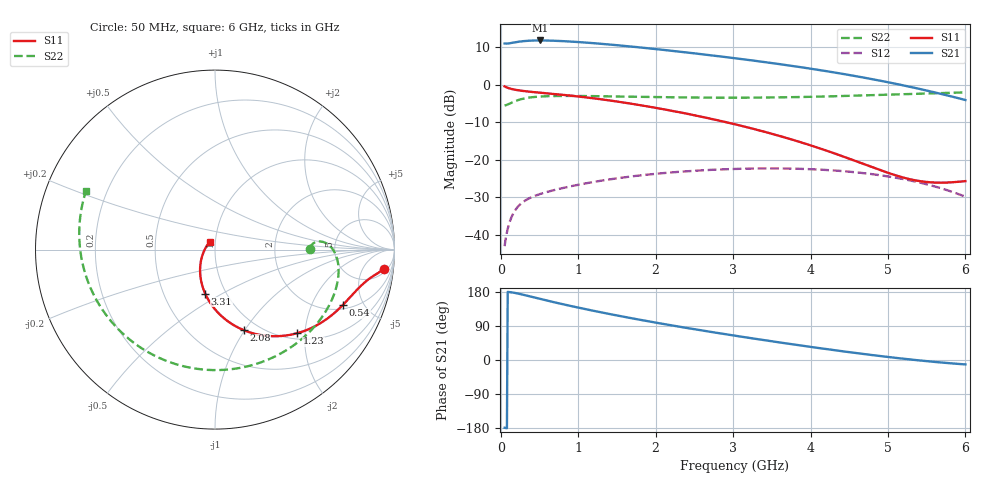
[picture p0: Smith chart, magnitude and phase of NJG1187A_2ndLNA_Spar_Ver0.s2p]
! Created Wed Mar 10 19:50:59 2021
# hz S ma R 50
! 2 Port Network Data from SP11.SP block
! freq  magS11  angS11  magS21  angS21  magS12  angS12  magS22  angS22
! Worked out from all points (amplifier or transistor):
!   596 points, 50 MHz to 6 GHz, reference 50 ohm
!   highest |S21| = 11.8 dB at 510 MHz (marker M1)
!   |S21| within 3 dB of that: start of sweep to 2.316 GHz
!   unconditionally stable (mu >= 1): start of sweep to end of sweep
!   at 1.04 GHz: K = 1.07, MAG = 17.2 dB, |S12| = -26.5 dB
!   at 3.03 GHz: K = 1.55, MAG = 10.4 dB, |S12| = -22.4 dB
!   at 6 GHz: K = 9.29, MAG = 0.2 dB, |S12| = -29.8 dB
!   lowest NFmin = 1.65 dB at 950 MHz
!   S11 on the Smith chart (normalised r, x): 50 MHz: 7, -15; 540 MHz: 2.24, -3.47; 1.23 GHz: 1.12, -1.82; 2.08 GHz: 0.85, -0.99; 3.31 GHz: 0.80, -0.42; 6 GHz: 0.94, +0.08
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5e7  0.9488 -6.5  3.533 -178.8  0.007091 81.8  0.5277 0.5
1.2e8  0.8874 -9.8  3.565 179.1  0.01537 68.4  0.563 4.3
2e8  0.8516 -12.6  3.686 176.4  0.02231 58.2  0.6113 3.8
3.4e8  0.8134 -17.0  3.833 169.7  0.02971 47.9  0.6668 -1.4
5.1e8  0.7816 -22.4  3.878 161.1  0.03511 42.6  0.6957 -8.4
5.4e8  0.7766 -23.4  3.877 159.6  0.03591 42.0  0.6984 -9.6
7.9e8  0.7348 -31.5  3.805 147.7  0.04188 39.4  0.7082 -18.9
1.05e9  0.6877 -39.9  3.665 136.1  0.04762 37.8  0.7071 -27.9
1.23e9  0.6526 -45.6  3.547 128.5  0.0514 36.7  0.7037 -33.8
1.42e9  0.6138 -51.4  3.413 120.7  0.05519 35.3  0.699 -40.0
1.61e9  0.5741 -57.1  3.273 113.3  0.05873 33.8  0.694 -46.2
2.04e9  0.484 -69.4  2.95 97.3  0.06571 29.9  0.6831 -60.3
2.08e9  0.4757 -70.5  2.92 95.8  0.06628 29.6  0.6821 -61.6
2.55e9  0.3825 -83.0  2.577 79.6  0.07197 24.8  0.6739 -77.6
3.03e9  0.2962 -95.4  2.246 64.0  0.07566 19.6  0.6713 -94.9
3.31e9  0.2508 -102.6  2.062 55.2  0.0767 16.4  0.6732 -105.4
3.65e9  0.201 -111.8  1.847 44.9  0.07669 12.3  0.6792 -118.4
4.02e9  0.1536 -122.6  1.622 34.0  0.07491 7.8  0.6902 -132.9
4.53e9  0.1008 -141.0  1.329 19.9  0.06909 1.8  0.7121 -152.8
5.01e9  0.06663 -165.9  1.073 7.8  0.05992 -2.9  0.7374 -171.0
5.49e9  0.05079 159.5  0.841 -2.9  0.04755 -5.2  0.7638 172.0
6e9  0.05208 125.6  0.6255 -11.7  0.03229 0.1  0.7897 155.4
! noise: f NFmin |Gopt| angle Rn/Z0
5e+07  2.091  0.8185  9.246  2.509
7.1e+08  1.661  0.3996  34.02  0.4175
1.37e+09  1.668  0.3584  54.91  0.3413
2.03e+09  1.745  0.3313  80.32  0.278
2.69e+09  1.885  0.3117  109.5  0.2166
3.35e+09  2.111  0.3057  140.8  0.1697
4.01e+09  2.466  0.3132  171  0.1563
4.67e+09  3.015  0.3248  -162.4  0.2008
5.33e+09  3.863  0.3278  -140  0.3395
6e+09  5.186  0.3122  -121.1  0.6453
